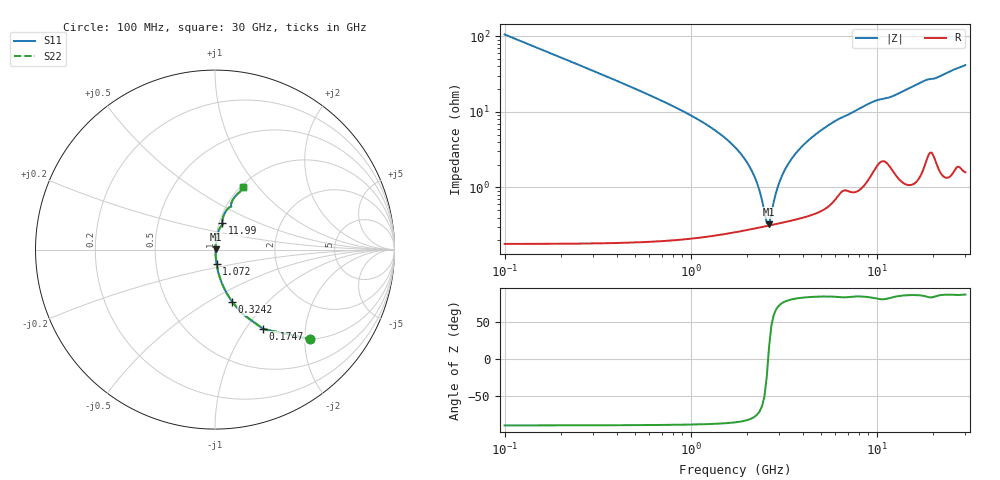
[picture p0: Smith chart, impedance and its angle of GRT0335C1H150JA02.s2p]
!Murata Part Number: GRT0335C1H150JA02
!These Parameters are Measured in Series Mode Connection
!Data Generated on Jun 19, 2026
!  o--ll--o
!Port1  Port2
!  o------o
!Operation Temp=25[degC], DC Bias Voltage=0[V]
!Freq. Start=100[MHz] Stop=30[GHz] 401[Steps]
# Hz S RI R 50
!Freq.(Hz) S11(Real) S11(Imag) S21(Real) S21(Imag) S12(Real) S12(Imag) S22(Real) S22(Imag)
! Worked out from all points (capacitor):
!   401 points, 100 MHz to 30 GHz, reference 50 ohm
!   read as one part in series: C = 15 pF near 249.5 MHz
!   lowest |Z| = 328 mohm at 2.642 GHz (marker M1)
!   series resonance near 2.611 GHz, so ESL is about 250 pH
!   S11 on the Smith chart (normalised r, x): 100 MHz: 1.00, -2.12; 174.8 MHz: 1.00, -1.21; 324.2 MHz: 1.00, -0.64; 1.072 GHz: 1.00, -0.16; 11.99 GHz: 1.04, +0.32; 30 GHz: 1.03, +0.83
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1e8  0.5288 -0.4983  0.4712 0.4983  0.4712 0.4983  0.5288 -0.4983
1.7475e8  0.2682 -0.4415  0.7318 0.4415  0.7318 0.4415  0.2682 -0.4415
3.2425e8  0.0953 -0.2908  0.9047 0.2908  0.9047 0.2908  0.0953 -0.2908
6.2325e8  0.0268 -0.1557  0.9732 0.1557  0.9732 0.1557  0.0268 -0.1557
1.07175e9  0.00878 -0.0811  0.9912 0.0811  0.9912 0.0811  0.00878 -0.0811
1.96875e9  0.00323 -0.0229  0.9968 0.0229  0.9968 0.0229  0.00323 -0.0229
2.26775e9  0.00302 -0.0113  0.997 0.0113  0.997 0.0113  0.00302 -0.0113
2.492e9  0.00305 -0.00371  0.997 0.00371  0.997 0.00371  0.00305 -0.00371
2.6415e9  0.00313 0.000947  0.9969 -0.000947  0.9969 -0.000947  0.00313 0.000947
2.71625e9  0.00318 0.00318  0.9968 -0.00318  0.9968 -0.00318  0.00318 0.00318
2.9405e9  0.0034 0.00954  0.9966 -0.00954  0.9966 -0.00954  0.0034 0.00954
3.09e9  0.00358 0.0135  0.9964 -0.0135  0.9964 -0.0135  0.00358 0.0135
3.46375e9  0.00414 0.0229  0.9959 -0.0229  0.9959 -0.0229  0.00414 0.0229
4.1365e9  0.00551 0.038  0.9945 -0.038  0.9945 -0.038  0.00551 0.038
5.10825e9  0.00831 0.0578  0.9917 -0.0578  0.9917 -0.0578  0.00831 0.0578
6.45375e9  0.0153 0.0814  0.9847 -0.0814  0.9847 -0.0814  0.0153 0.0814
1.01165e10  0.038 0.1341  0.962 -0.1341  0.962 -0.1341  0.038 0.1341
1.198525e10  0.0405 0.1489  0.9595 -0.1489  0.9595 -0.1489  0.0405 0.1489
1.505e10  0.0507 0.195  0.9493 -0.195  0.9493 -0.195  0.0507 0.195
2.005825e10  0.0905 0.2412  0.9095 -0.2412  0.9095 -0.2412  0.0905 0.2412
2.50665e10  0.1182 0.303  0.8818 -0.303  0.8818 -0.303  0.1182 0.303
3e10  0.1578 0.346  0.8422 -0.346  0.8422 -0.346  0.1578 0.346
